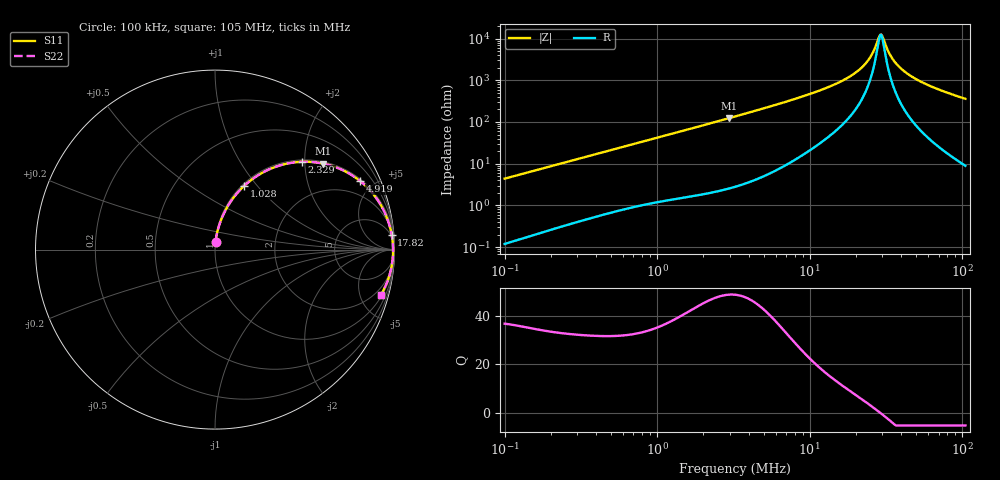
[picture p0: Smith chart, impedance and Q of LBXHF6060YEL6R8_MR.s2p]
! LBXHF6060YEL6R8_MR  S-PARAMETER MODEL  ( General Type )
! Model Generated by TAIYO YUDEN Corporation (http://www.ty-top.com)
! Version 1.0
! TAIYO YUDEN Control No. 200217NI43SB-FBB
! Copyright(c) 2020 TAIYO YUDEN CO.,LTD. All Rights Reserved.
! Product Description (link to TY-COMPAS)
! https://ds.yuden.co.jp/TYCOMPAS/or/detail?pn=LBXHF6060YEL6R8MMR&u=M
! Products Name : Inductors
! Characteristics :
!  Inductance : 6.8 uH , SRF(min) : 20 MHz , DC Resistance(max) : 0.052 Ohm
!  Rated Current : Saturation :5100 mA , Temp Rise : 1900 mA
!  Case Size : 6.0 x 6.0 / 0.236 x 0.236 [mm/inch] , Thickness : 4.5 / 0.177 [mm/inch]
!  (Conditions: Temperature = 25 degC , DC Bias Current/Voltage = 0A / 0V)
! External Node Assignments :
!  1  o---GGG---o  2
! GND o---------o GND
! Frequency Range : 0.1MHz  -  105.0131MHz  [ 402 STEP ]
# MHz S RI R 50
! Freq[MHz].  S11 Real  S11 Imag  S21 Real  S21 Imag  S12 Real  S12 Imag  S22 Real  S22 Imag
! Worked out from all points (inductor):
!   401 points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, 100 kHz to 105 MHz, reference 50 ohm
!   read as one part in series: L = 6.95 uH near 103.5 kHz
!   highest Q = 48.6 at 2.971 MHz (marker M1), where L = 6.65 uH
!   self-resonance near 28.99 MHz
!   S11 on the Smith chart (normalised r, x): 100 kHz: 1.00, +0.09; 1.028 MHz: 1.02, +0.86; 2.329 MHz: 1.04, +1.94; 4.919 MHz: 1.10, +4.18; 17.82 MHz: 3, +23; 105 MHz: 1.18, -7.22
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0.1  0.0031 0.0436  0.9969 -0.0436  0.9969 -0.0436  0.0031 0.0436
0.32067  0.0226 0.134  0.9774 -0.134  0.9774 -0.134  0.0226 0.134
0.620978  0.0712 0.242  0.9288 -0.242  0.9288 -0.242  0.0712 0.242
1.028292  0.1633 0.3558  0.8367 -0.3558  0.8367 -0.3558  0.1633 0.3558
1.507596  0.2877 0.4405  0.7123 -0.4405  0.7123 -0.4405  0.2877 0.4405
2.328695  0.4851 0.4893  0.5149 -0.4893  0.5149 -0.4893  0.4851 0.4893
2.970682  0.6042 0.4788  0.3958 -0.4788  0.3958 -0.4788  0.6042 0.4788
3.297424  0.6529 0.4659  0.3471 -0.4659  0.3471 -0.4659  0.6529 0.4659
4.919221  0.8085 0.382  0.1915 -0.382  0.1915 -0.382  0.8085 0.382
10.39154  0.952 0.1917  0.048 -0.1917  0.048 -0.1917  0.952 0.1917
17.81666  0.9841 0.0837  0.0159 -0.0837  0.0159 -0.0837  0.9841 0.0837
21.20106  0.9887 0.0536  0.0113 -0.0536  0.0113 -0.0536  0.9887 0.0536
23.94579  0.9907 0.0332  0.00929 -0.0332  0.00929 -0.0332  0.9907 0.0332
25.67093  0.9915 0.0217  0.00852 -0.0217  0.00852 -0.0217  0.9915 0.0217
28.00317  0.9921 0.00742  0.00794 -0.00742  0.00794 -0.00742  0.9921 0.00742
28.99435  0.9922 0.00172  0.00783 -0.00172  0.00783 -0.00172  0.9922 0.00172
30.02062  0.9922 -0.00399  0.00778 0.00399  0.00778 0.00399  0.9922 -0.00399
33.32256  0.9919 -0.0212  0.00805 0.0212  0.00805 0.0212  0.9919 -0.0212
38.29686  0.9906 -0.0445  0.00941 0.0445  0.00941 0.0445  0.9906 -0.0445
48.01242  0.9856 -0.0842  0.0144 0.0842  0.0144 0.0842  0.9856 -0.0842
66.81326  0.9703 -0.1486  0.0297 0.1486  0.0297 0.1486  0.9703 -0.1486
105.0131  0.9233 -0.254  0.0767 0.254  0.0767 0.254  0.9233 -0.254
